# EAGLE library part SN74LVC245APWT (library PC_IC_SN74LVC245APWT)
OCTAL BUS TRANSCEIVER WITH 3-STATE OUTPUTS
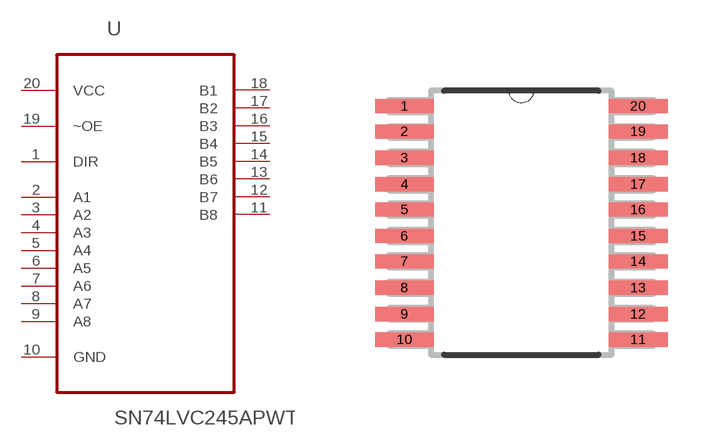
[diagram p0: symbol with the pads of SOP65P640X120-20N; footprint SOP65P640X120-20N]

Designator prefix U

## SN74LVC245APWT (Availability: Unavailable; Description: Octal Bus Transceiver With 3-State Outputs 20-TSSOP -40 to 125; MF: Texas Instruments; MP: SN74LVC245APWT; Package: TSSOP-20 Texas Instruments; Price: None)  [SOP65P640X120-20N]
1  DIR  in
2  A1
3  A2
4  A3
5  A4
6  A5
7  A6
8  A7
9  A8
10  GND  pas
11  B8
12  B7
13  B6
14  B5
15  B4
16  B3
17  B2
18  B1
19  ~OE  in
20  VCC  pwr

## Footprint SOP65P640X120-20N (pad centres in mm)
smd 1.473 x 0.356: 1 -2.921,2.921; 2 -2.921,2.286; 3 -2.921,1.626; 4 -2.921,0.965; 5 -2.921,0.33; 6 -2.921,-0.33; 7 -2.921,-0.965; 8 -2.921,-1.626; 9 -2.921,-2.286; 10 -2.921,-2.921; 11 2.921,-2.921; 12 2.921,-2.286; 13 2.921,-1.626; 14 2.921,-0.965; 15 2.921,-0.33; 16 2.921,0.33; 17 2.921,0.965; 18 2.921,1.626; 19 2.921,2.286; 20 2.921,2.921

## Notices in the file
This work is licensed under a Creative Commons Attribution-ShareAlike 4.0 International License (CC BY-SA) with Design Exception 1.0
